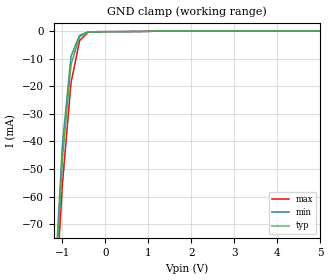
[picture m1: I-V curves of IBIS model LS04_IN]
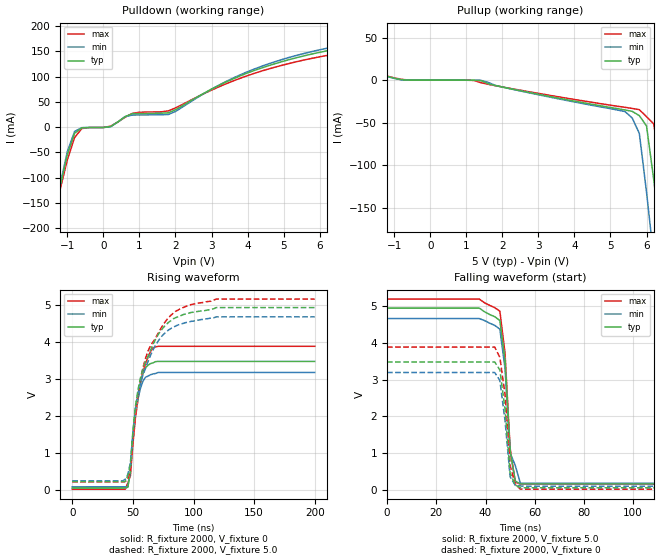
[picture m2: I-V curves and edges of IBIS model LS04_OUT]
|   TEXAS INSTRUMENTS INCORPORATED
|   Standard Linear and Logic
|   IBIS Model of SN74LS04
|   HEX INVERTERS
|   SOIC 14-pin (D), SOP 14-pin (NS), P-DIP 14-pin (N)
[IBIS Ver]   3.2
[Comment Char]  |_char
[File Name]   sn74ls04.ibs
[File Rev]   3.2 | c_die
[Date]   11/11/04
[Source]   File originated at Texas Instruments, Inc.
[Notes]   The following is a sample IBIS file for the SN74LS04.
   - FILE REV HISTORY
   - 3.2 Re-Release IBIS file on 11/11/04
   - Power clamp data deleted as there is no power-clamp diode.
   - All test data contained in this file are derived from
   actual measurement.
   - The measurement used NS package.
   - We have data across voltage and temperature, but not across
   process.
|   - File created by Nobuhisa Ohtsubo, TIJ SLL Product Engineering.
[Disclaimer] Property of Texas Instruments Incorporated.  Unauthorized
   reproduction and/or distribution is strictly prohibited.
   This product is protected under copyright law.
   Created 2000, (C) Copyright 2000, Texas Instruments Inc.,
   All Rights Reserved.
   UNLESS THERE IS A SIGNED, WRITTEN AGREEMENT TO THE
   CONTRARY, TEXAS INSTRUMENTS () IS PROVIDING THE IBIS
   MODELS  AND WITHOUT ANY WARRANTY, EXPRESSED OR
   IMPLIED.  TI assumes no liability for:
   1) the accuracy of the IBIS models provided to your
   company;
   2) the proper functioning of these IBIS Models in your
   design or for any resulting applications; or
   3) infringement of patents, copyrights or intellectual
   property rights resulting from your use of these IBIS
   models.
   TI provides IBIS Models as a service to our customers.
   You and your company shall not distribute, sell or give
   these models to anyone else without prior written
   permission from TI.
   TI reserves the right to make changes to our products or
   to discontinue any semiconductor product or service
   without notice, and advises our customers to obtain the
   latest version of relevant information to verify, before
   placing orders, that the information being relied on is
   current.
   Please be aware that your receipt and use of the IBIS
   information provided shall serve as acceptance of these
   terms and conditions.  If you do not accept these terms,
   you should return or destroy the IBIS models and any
   other accompanying information immediately.
|   Component LS04_D
[Component]   LS04_D
[Manufacturer]  Texas Instruments, Inc.
[Package]
|   typ   min   max
R_pkg   0.031   0.028   0.034
L_pkg   3.109nH   2.462nH   3.889nH
C_pkg   0.473pF   0.363pF   0.628pF
[Pin]   signal_name   model_name   R_pin   L_pin   C_pin
1   1A   LS04_IN   0.033   3.854nH   0.622pF
2   1Y   LS04_OUT   0.032   3.188nH   0.473pF
3   2A   LS04_IN   0.028   2.462nH   0.377pF
4   2Y   LS04_OUT   0.031   2.596nH   0.363pF
5   3A   LS04_IN   0.028   2.521nH   0.372pF
6   3Y   LS04_OUT   0.034   3.250nH   0.476pF
7   GND   GND   0.034   3.889nH   0.628pF
8   4Y   LS04_OUT   0.034   3.889nH   0.628pF
9   4A   LS04_IN   0.034   3.250nH   0.476pF
10   5Y   LS04_OUT   0.028   2.521nH   0.372pF
11   5A   LS04_IN   0.031   2.596nH   0.364pF
12   6Y   LS04_OUT   0.028   2.462nH   0.377pF
13   6A   LS04_IN   0.032   3.188nH   0.473pF
14   VCC   POWER   0.033   3.854nH   0.622pF
|   Component LS04_NS
[Component]   LS04_NS
[Manufacturer]  Texas Instruments, Inc.
[Package]
|   typ   min   max
R_pkg   0.045   0.039   0.054
L_pkg   3.796nH   2.561nH   4.952nH
C_pkg   0.528pF   0.288pF   0.710pF
[Pin]   signal_name   model_name   R_pin   L_pin   C_pin
1   1A   LS04_IN   0.047   4.867nH   0.706pF
2   1Y   LS04_OUT   0.051   4.083nH   0.592pF
3   2A   LS04_IN   0.041   2.915nH   0.376pF
4   2Y   LS04_OUT   0.039   2.561nH   0.288pF
5   3A   LS04_IN   0.041   3.101nH   0.430pF
6   3Y   LS04_OUT   0.047   4.047nH   0.589pF
7   GND   GND   0.051   4.909nH   0.700pF
8   4Y   LS04_OUT   0.045   4.784nH   0.694pF
9   4A   LS04_IN   0.054   4.176nH   0.597pF
10   5Y   LS04_OUT   0.039   3.287nH   0.449pF
11   5A   LS04_IN   0.039   2.586nH   0.294pF
12   6Y   LS04_OUT   0.040   2.802nH   0.371pF
13   6A   LS04_IN   0.049   4.080nH   0.593pF
14   VCC   POWER   0.052   4.952nH   0.710pF
|   Component LS04_N
[Component]   LS04_N
[Manufacturer]   Texas Instruments, Inc.
[Package]
|   typ   min   max
R_pkg   4.500e-02   3.700e-02   6.300e-02
L_pkg   5.407e-09   3.922e-09   6.942e-09
C_pkg   3.890e-13   2.050e-13   6.040e-13
[Pin]   signal_name   model_name   R_pin   L_pin   C_pin
1   1A   LS04_IN   6.300e-02   6.942e-09   6.040e-13
2   1Y   LS04_OUT   3.700e-02   6.200e-09   4.060e-13
3   2A   LS04_IN   4.200e-02   4.389e-09   3.220e-13
4   2Y   LS04_OUT   3.800e-02   3.922e-09   2.050e-13
5   3A   LS04_IN   3.900e-02   4.301e-09   2.980e-13
6   3Y   LS04_OUT   3.800e-02   5.329e-09   3.560e-13
7   GND   GND   5.300e-02   6.510e-09   5.440e-13
8   4Y   LS04_OUT   5.300e-02   6.437e-09   5.390e-13
9   4A   LS04_IN   3.900e-02   5.352e-09   3.470e-13
10   5Y   LS04_OUT   4.200e-02   4.473e-09   2.970e-13
11   5A   LS04_IN   4.400e-02   4.326e-09   2.250e-13
12   6Y   LS04_OUT   4.200e-02   4.295e-09   2.800e-13
13   6A   LS04_IN   4.200e-02   6.318e-09   4.180e-13
14   VCC   POWER   6.100e-02   6.900e-09   6.030e-13
| Models and submodels in the file (2): LS04_IN (Input), LS04_OUT (Output)
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|   Model LS04_IN
[Model]   LS04_IN
Model_type  Input
Polarity   Inverting
Vinl = 0.8
Vinh = 2.0
| variable   typ   min   max
C_comp   1.33pf   1.00pf   1.66pf
[Temperature Range]   25   0   70
[Voltage Range]   5.0   4.75   5.25
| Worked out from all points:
|   GND clamp passes 1 mA (typ) near -0.49 V on its own axis
[GND Clamp]
|   Voltage   I(typ)   I(min)   I(max)
-5V       -1.511A    -1.595A    -1.368A
-1.2V     -103mA     -97.59mA   -108.2mA
-1V       -46.17mA   -41.15mA   -55.44mA
-800mV    -12.1mA    -9.107mA   -18.75mA
-600mV    -1.943mA   -1.524mA   -3.398mA
-400mV    -278uA     -260.1uA   -441.6uA
-200mV    -233.9uA   -241.2uA   -211uA
5V        14.74nA    12.93nA    37.82nA
|   Model LS04_OUT
[Model]   LS04_OUT
Model_type  Output
Polarity   Non-Inverting
Vmeas = 1.3v
Cref = 15pf
Rref = 2000
Vref = 0V
| variable   typ   min   max
C_comp   5.8pf   4.35pf   7.25pf
[Temperature Range]   25   0   70
[Voltage Range]   5.0   4.75   5.25
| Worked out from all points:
|   slope of the pulldown table from 0 to 0.75 V, typ, clamps not added: 29 ohm
|   slope of the pullup table from 0 to 0.75 V, typ, clamps not added: 29.7 kohm
|   rising waveform, R_fixture 2000, V_fixture 0: 20-80 % time 7.11ns typ, 6.52ns min, 8.96ns max; typ from 0.052 V to 3.47 V
|   falling waveform, R_fixture 2000, V_fixture 5.0: 20-80 % time 2.91ns typ, 2.91ns min, 2.9ns max; typ from 4.95 V to 0.156 V
|   rising waveform, R_fixture 2000, V_fixture 5.0: 20-80 % time 18.4ns typ, 17.7ns min, 20.1ns max; typ from 0.223 V to 4.93 V
|   falling waveform, R_fixture 2000, V_fixture 0: 20-80 % time 2.9ns typ, 2.9ns min, 3.01ns max; typ from 3.48 V to 0.051 V
[Pulldown]
|   Voltage   I(typ)   I(min)   I(max)
-5V       -1.565A    -1.648A    -1.412A
-1.6V     -264.6mA   -269.4mA   -255.5mA
-1.4V     -189mA     -189mA     -187.9mA
-1V       -54.56mA   -48.37mA   -64.76mA
-800mV    -12.27mA   -8.526mA   -20.77mA
-600mV    -1.349mA   -1mA       -2.903mA
200mV     1.168mA    720.9uA    1.873mA
800mV     26.61mA    23.94mA    27.32mA
1.8V      28.38mA    25.05mA    32.13mA
3.6V      95.69mA    97.34mA    91.56mA
5.4V      138.4mA    143mA      130.4mA
10V       193.8mA    200.3mA    179.9mA
[Pullup]
|   Voltage   II(typ)   I(min)   I(max)
-5V       57.51mA    60.79mA    50.84mA
-1V       2.321mA    2.072mA    2.732mA
1.4V      -488.2uA   -178.4uA   -2.918mA
2.4V      -11.59mA   -11.82mA   -11.08mA
5.4V      -35.02mA   -36.85mA   -31.9mA
5.6V      -36.64mA   -44.29mA   -33.21mA
5.8V      -41.68mA   -62.59mA   -34.69mA
6V        -53.84mA   -131.7mA   -42.93mA
6.2V      -116.9mA   -209mA     -51.48mA
6.4V      -188.9mA   -289.9mA   -107.2mA
6.6V      -265.1mA   -372.3mA   -171.2mA
10V       -1.595A    -1.785A    -1.338A
[Ramp]
| variable   typ   min   max
dV/dt_r  1.956E+00/7.506E-09  1.764E+00/7.055E-09  2.204E+00/8.789E-09
dV/dt_f  2.820E+00/1.526E-09  2.658E+00/1.594E-09  2.982E+00/1.435E-09
R_load=2000
[Rising Waveform]
R_fixture = 2000
V_fixture = 0
V_fixture_min = 0
V_fixture_max = 0
C_fixture = 0pf
L_fixture = 0nH
|   Time   V(typ)   V(min)   V(max)
0s        51.98mV    83.41mV    20.04mV
43.75ns   52.44mV    84.19mV    20.18mV
45.83ns   72.5mV     86.19mV    189.7mV
47.92ns   507.3mV    483.6mV    378.3mV
50ns      1.494V     1.469V     1.233V
52.08ns   2.151V     2.099V     1.945V
56.25ns   2.906V     2.754V     2.858V
60.42ns   3.302V     3.047V     3.419V
66.67ns   3.437V     3.136V     3.844V
200ns     3.474V     3.176V     3.883V
[Falling Waveform]
R_fixture = 2000
V_fixture = 5.0
V_fixture_min = 4.75
V_fixture_max = 5.25
C_fixture = 0pf
L_fixture = 0nH
|   Time   V(typ)   V(min)   V(max)
0s        4.951V     4.666V     5.198V
37.5ns    4.951V     4.666V     5.198V
39.58ns   4.853V     4.612V     5.096V
43.75ns   4.717V     4.481V     4.963V
45.83ns   4.612V     4.377V     4.868V
47.92ns   3.541V     3.309V     3.73V
50ns      1.058V     992.8mV    1.131V
52.08ns   235.4mV    661.4mV    208.1mV
54.17ns   156mV      172.4mV    146.7mV
200ns     156mV      172.4mV    146.7mV
[Rising Waveform]
R_fixture = 2000
V_fixture = 5.0
V_fixture_min = 4.75
V_fixture_max = 5.25
C_fixture = 0pf
L_fixture = 0nH
|   Time   V(typ)   V(min)   V(max)
0s        223.1mV    246.9mV    210mV
45.83ns   378.5mV    420.9mV    308.3mV
47.92ns   676.2mV    731.1mV    483.5mV
52.08ns   2.26V      2.217V     2.067V
56.25ns   3.031V     2.886V     2.983V
60.42ns   3.471V     3.287V     3.557V
72.92ns   4.296V     4.122V     4.358V
85.42ns   4.659V     4.433V     4.834V
118.8ns   4.931V     4.679V     5.16V
200ns     4.931V     4.679V     5.16V
[Falling Waveform]
R_fixture = 2000
V_fixture = 0
V_fixture_min = 0
V_fixture_max = 0
C_fixture = 0pf
L_fixture = 0nH
|   Time   V(typ)   V(min)   V(max)
0s        3.482V     3.195V     3.889V
43.75ns   3.482V     3.195V     3.889V
45.83ns   3.265V     2.978V     3.609V
47.92ns   2.207V     1.891V     2.605V
50ns      451.3mV    348.9mV    663.8mV
52.08ns   125.5mV    120.8mV    139.2mV
54.17ns   52.31mV    100.8mV    14.21mV
56.25ns   51.04mV    92.44mV    13.22mV
200ns     51.04mV    92.44mV    13.22mV
